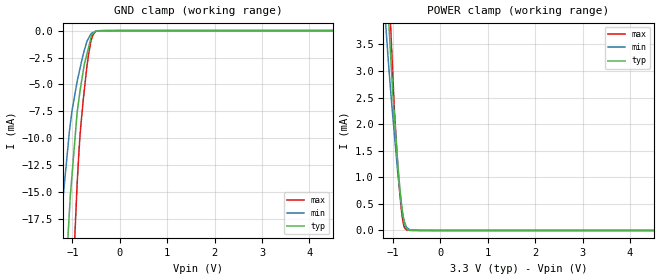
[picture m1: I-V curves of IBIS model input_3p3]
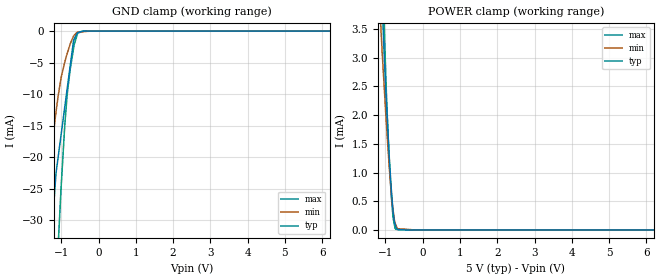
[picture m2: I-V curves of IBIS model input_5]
|Texas Instruments Incorporated
| 14-Bit, Single Channel, Parallel Interface,
| Multiplying Digital-to-Analog Converter
| Marketing part#   Digital Voltage Range   Package-type   #pins
| DAC8806IDB   2.7V - 5.5V   SSOP   28
| DAC8806IDBG4   2.7V - 5.5V   SSOP   28
| DAC8806IDBR   2.7V - 5.5V   SSOP   28
| DAC8806IDBRG4   2.7V - 5.5V   SSOP   28
[IBIS Ver]   3.2
[File name]   dac8806.ibs
|SIMDE Ver   V3.0 - 201101 - RHL4 - Build 453
[File Rev]   1.0
[Date]   4/19/2011
[Source]
| Texas Instruments Incorporated.
| Analog-eLab Design Center, HPA
| 12500 TI Blvd
| Dallas, TX -75243
| e-mail: elab_ibis@list.ti.com
| -Model generated from simulations in TISPICE
[Notes]   Revision History:
| Rev 1.0: 4/19/2011
| - Initial version of the model
| - Model generated from simulations in TISPICE
| - Model matched to SPICE simulation
| - C_comp although listed in numerical order of value are
|   obtained from varying PVT conditions. For PVT conditions for
|   each specific value refer the buffer description under
|   respective [Model]. IBIS model user is responsible for using
|   appropriate C_comp to simulate for Signal Integrity.
| - Model names with a trailing _3p3 contains
|   the model for 3.3V [3.0V and 3.6V]. Model names with trailing _5
|   contains the model for 5.0V [4.5V and 5.5V] operation.
| - Relative part of DAC8820.
[Disclaimer]
| This model is designed as an aid for customers of Texas Instruments.
| TI and its licensors and suppliers make no warranties, either expressed
| or implied, with respect to this  model, including the warranties of
| merchantability or fitness for a particular purpose. The model is
| provided solely on an "as is" basis. The entire risk as to its quality
| and performance is with the customer.
[Copyright]
 (C) Copyright 2011 Texas Instruments Incorporated.All rights reserved.
|   DAC8806
[Component]   DAC8806
[Manufacturer]   TI
[Package]   |28 SSOP   -  DB package
|   typ   min   max
R_pkg   0.06167   0.03749   0.07954
L_pkg   4.12587nH   2.60825nH   6.96328nH
C_pkg   0.84568pF   0.45801pF   1.45149pF
[Pin]  signal_name   model_name   R_pin   L_pin   C_pin
1   REF   TERM   0.04262   6.28347nH  1.34440pF
2   RCOM   TERM   0.03945   5.16122nH  1.30353pF
3   R1   TERM   0.03749   4.42095nH  1.05211pF
4   ROFS   TERM   0.07479   3.76378nH  0.70623pF
5   RFB   TERM   0.06774   3.07944nH  0.54451pF
6   IOUT   TERM   0.06351   2.75581nH  0.47395pF
7   AGND   GND   0.03267   2.36889nH  0.49875pF
8   LDAC   INPUT   0.05870   2.60825nH  0.45801pF
9   _WR   INPUT   0.06002   2.64965nH  0.46742pF
10   D13   INPUT   0.06372   2.95868nH  0.53563pF
11   D12   INPUT   0.06991   3.61781nH  0.68970pF
12   D11   INPUT   0.06015   4.27605nH  0.95491pF
13   D10   INPUT   0.05971   5.03572nH  1.20368pF
14   D9   INPUT   0.06461   6.96328nH  1.45149pF
15   D8   INPUT   0.06472   6.71543nH  1.40135pF
16   D7   INPUT   0.06166   5.14407nH  1.22804pF
17   D6   INPUT   0.06280   4.40930nH  0.96971pF
18   D5   INPUT   0.06918   3.55292nH  0.67200pF
19   D4   INPUT   0.06349   2.76278nH  0.48910pF
20   D3   INPUT   0.06026   2.65742nH  0.46903pF
21   D2   INPUT   0.05895   2.61631nH  0.46672pF
22   DGND   GND   0.02339   2.29964nH  0.54786pF
23   VDD   POWER   0.03508   2.53436nH  0.52659pF
24   D1   INPUT   0.07126   3.19056nH  0.55504pF
25   D0   INPUT   0.07954   3.91552nH  0.71548pF
26   NC   NC   0.07105   4.84051nH  1.02565pF
27   NC   NC   0.06020   5.20445nH  1.24563pF
28   _RST   INPUT   0.06417   6.35669nH  1.29857pF
|   Model Selectors
[Model Selector] INPUT
input_3p3  3.3V digital input
input_5   5.0V digital input
[Model Selector] TERM
term_3-3V  3.3V nominal termination
term_5-0V  5.0V nominal termination
[Model]  term_3-3V
Model_type Terminator
C_comp   1.0e-20F  1.0e-20F  1.0e-20F
|   typ   min   max
[Voltage Range]   3.3V   3.0V   3.6V
[POWER Clamp Reference]   3.3V   3.0V   3.6V
[GND Clamp Reference]   0V   0V   0V
|Ambient Temperature   25   85   -40
|Junction Temperature
[Temperature Range]   25   85   -40
[Model]  term_5-0V
Model_type Terminator
C_comp   1.0e-20F  1.0e-20F  1.0e-20F
|   typ   min   max
[Voltage Range]   5.0V   4.5V   5.5V
[POWER Clamp Reference]   5.0V   4.5V   5.5V
[GND Clamp Reference]   0V   0V   0V
|Ambient Temperature   25   85   -40
|Junction Temperature
[Temperature Range]   25   85   -40
| Models and submodels in the file (4): input_3p3 (Input), input_5 (Input), term_3-3V (Terminator), term_5-0V (Terminator)
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|   input_3p3 Model
[Model]   input_3p3
Model_type   Input
Vinl = 0.6
Vinh = 2.1
|   typ   min   max
|   (nom PVT)   (Fast PVT)   (slow PVT)
|C_comp from frequency method(F=25MHz)
|Average
|C_comp   3.212e-12   3.013e-12   3.421e-12
|C_comp from L-C Tank method(L=1nH)
|Resonant Frequency(Hz)   3.640e9   3.850e9   3.420e9
C_comp   1.914e-12   1.711e-12   2.168e-12
| Where nom  PVT is Nominal Process,  3.3V,  25C
|   Fast PVT is Strong Process,   3.6V,  -40C
|   Slow PVT is Weak Process,   3V,  85C
[Voltage Range]   3.3   3   3.6
|Ambient Temperature   25   85   -40
|Junction Temperature
[Temperature Range]   25   85   -40
[Power Clamp Reference]   3.3   3   3.6
[GND Clamp Reference]   0   0   0
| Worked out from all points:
|   GND clamp passes 1 mA (typ) near -0.62 V on its own axis
|   POWER clamp passes 1 mA (typ) near -0.87 V on its own axis
[GND Clamp]
|   Voltage   I(typ)   I(min)   I(max)
-3.3V     -272.4mA   -193.6mA   -368.1mA
-1.432V   -48.92mA   -29.38mA   -81.72mA
-1.248V   -31.68mA   -18.19mA   -56.02mA
-1.141V   -23.02mA   -13.08mA   -41.16mA
-1.059V   -16.68mA   -9.306mA   -31.32mA
-1.008V   -13.55mA   -7.511mA   -25.21mA
-897.6mV  -7.599mA   -4.727mA   -14.26mA
-824.4mV  -5.259mA   -3.271mA   -9.082mA
-698.4mV  -2.298mA   -1.114mA   -3.607mA
-604.8mV  -666.8uA   -298.6uA   -961.2uA
-498mV    -52.41uA   -37.63uA   -67.47uA
6.6V      0A         0A         0A
[POWER Clamp]
|   Voltage   I(typ)   I(min)   I(max)
-3.3V     49.6mA     41.68mA    60.04mA
-1.152V   5.063mA    3.882mA    6.177mA
-1.089V   3.945mA    3.099mA    4.757mA
-1.051V   3.354mA    2.669mA    3.909mA
-1.035V   3.101mA    2.485mA    3.588mA
-968.4mV  2.155mA    1.808mA    2.268mA
-896.4mV  1.251mA    1.078mA    1.18mA
-871.2mV  978.9uA    873uA      880.2uA
-792mV    301.3uA    309.6uA    189uA
-712.8mV  32.6uA     63.65uA    8.2uA
-591mV    5.576uA    2.097uA    177.4nA
6.6V      0A         0A         0A
|   input_5 Model
[Model]   input_5
Model_type   Input
Vinl = 0.8
Vinh = 2.4
|   typ   min   max
|   (nom PVT)   (Fast PVT)   (slow PVT)
|C_comp from frequency method(F=25MHz)
|Average
|C_comp   3.104e-12   2.903e-12   3.316e-12
|C_comp from L-C Tank method(L=1nH)
|Resonant Frequency(Hz)   3.620e9   3.830e9   3.440e9
C_comp   1.935e-12   1.729e-12   2.143e-12
| Where nom  PVT is Nominal Process,  5V,  25C
|   Fast PVT is Strong Process,   5.5V,  -40C
|   Slow PVT is Weak Process,   4.5V,  85C
[Voltage Range]   5   4.5   5.5
|Ambient Temperature   25   85   -40
|Junction Temperature
[Temperature Range]   25   85   -40
[Power Clamp Reference]   5   4.5   5.5
[GND Clamp Reference]   0   0   0
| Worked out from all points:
|   GND clamp passes 1 mA (typ) near -0.63 V on its own axis
|   POWER clamp passes 1 mA (typ) near -0.87 V on its own axis
[GND Clamp]
|   Voltage   I(typ)   I(min)   I(max)
-5V       -488mA     -367.3mA   -630.2mA
-1.575V   -63.69mA   -39.01mA   -102.4mA
-1.375V   -43.29mA   -25.61mA   -73.01mA
-1.25V    -31.7mA    -18.61mA   -55.6mA
-1.14V    -22.51mA   -12.81mA   -41.13mA
-1.089V   -20.23mA   -10.5mA    -34.65mA
-999mV    -16.2mA    -7.23mA    -24.28mA
-913mV    -12.35mA   -5.086mA   -15.59mA
-841.5mV  -9.15mA    -3.558mA   -10.07mA
-670mV    -1.474mA   -783.5uA   -2.731mA
-571.5mV  -322.7uA   -167.7uA   -561.2uA
10V       0A         0A         0A
[POWER Clamp]
|   Voltage   I(typ)   I(min)   I(max)
-5V       84.94mA    72.38mA    102.3mA
-1.122V   4.536mA    3.516mA    5.485mA
-1.089V   3.974mA    3.099mA    4.738mA
-1.045V   3.224mA    2.611mA    3.777mA
-990mV    2.414mA    2.001mA    2.664mA
-913mV    1.448mA    1.238mA    1.399mA
-852.5mV  797.1uA    727.5uA    679.9uA
-797.5mV  336.7uA    354.9uA    221.1uA
-760mV    141.2uA    175.1uA    91.03uA
-715mV    35.14uA    78.03uA    9.046uA
-202.5mV  0A         0A         2.562uA
10V       0A         0A         0A
